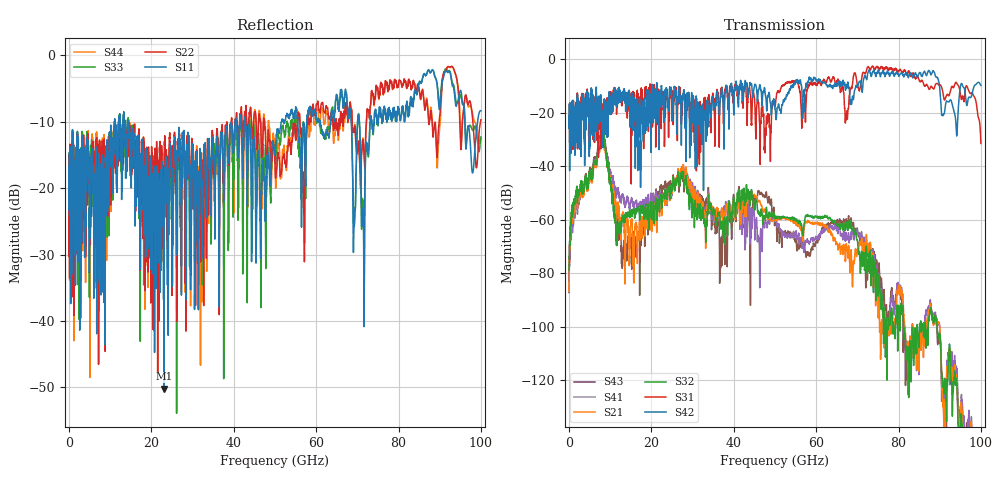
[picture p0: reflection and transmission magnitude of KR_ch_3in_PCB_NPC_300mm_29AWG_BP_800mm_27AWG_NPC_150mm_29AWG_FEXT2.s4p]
# GHz S RI R 45
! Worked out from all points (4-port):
!   4000 points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, 25 MHz to 100 GHz, reference 45 ohm
!   strongest paths, dB at 25 MHz, 25.02 GHz, 50.02 GHz, 75.03 GHz, 100 GHz:
!     S42: -21.2, -20.7, -18.6, -4.1, -9.8
!     S31: -21.2, -13.7, -17.5, -2.9, -31.4
!     S32: -78.9, -48.6, -59.7, -86.2, -145.6
!     S21: -86.8, -49.2, -60.4, -92.7, -148.4
!     S41: -87.3, -49.9, -60.3, -83.8, -139.9
!     S43: -87.1, -46.8, -59.7, -81.1, -139.8
!   lowest |S11| = -50.2 dB at 23.1 GHz (marker M1), VSWR 1.01, Z = 45 - j0.275 ohm
!   |S11| at or under -10 dB: start of sweep to 11.02 GHz; 14.38 GHz to 40.34 GHz (25.96 GHz wide, 94.9 % of centre); 42.82 GHz to 51.61 GHz (8.794 GHz wide, 18.6 % of centre)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
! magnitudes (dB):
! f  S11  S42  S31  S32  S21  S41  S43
! 25 MHz  -16.7  -21.2  -21.2  -78.9  -86.8  -87.3  -87.1
! 8 GHz  -16.0  -26.2  -24.8  -27.0  -28.7  -27.3  -25.6
! 13.22 GHz  -9.0  -11.8  -13.4  -59.6  -58.8  -51.9  -70.0
! 23.1 GHz  -50.2  -15.1  -20.0  -50.1  -50.6  -50.4  -47.1
! 47.8 GHz  -20.7  -14.2  -28.4  -57.8  -57.6  -60.8  -50.5
! 77.12 GHz  -9.8  -5.1  -2.8  -106.3  -108.2  -103.6  -96.7
! 100 GHz  -8.3  -9.8  -31.4  -145.6  -148.4  -139.9  -139.8
